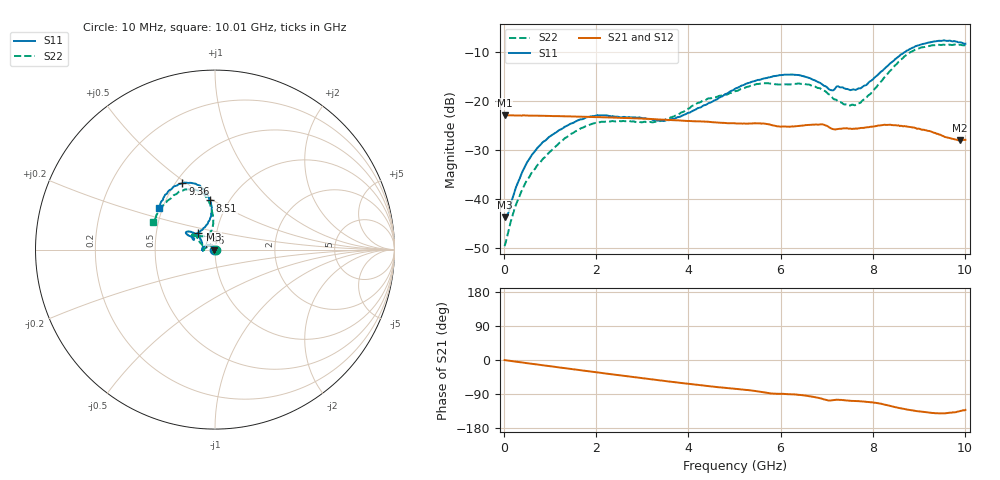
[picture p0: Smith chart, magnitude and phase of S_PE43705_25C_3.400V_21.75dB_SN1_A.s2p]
! Device ID: PE43705
! Serial: 1
! Insertion: A
! Impedance: 50 ohm
! Temp: 25C
! VDD: 3.400V
! Attenuation Step: 21.75dB
#  Hz  S  RI  R  50
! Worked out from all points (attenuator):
!   401 points, 10 MHz to 10.01 GHz, reference 50 ohm
!   highest |S21| = -22.82 dB at 10 MHz (marker M1); lowest = -28.0 dB at 9.885 GHz (marker M2)
!   lowest |S11| = -43.7 dB at 10 MHz (marker M3), VSWR 1.01, Z = 49.4 + j0.0459 ohm
!   |S11| at or under -10 dB: start of sweep to 8.682 GHz
!   |S22| runs from -49.6 to -8.4 dB; largest |S21 - S12| = 0.00086
!   S11 on the Smith chart (normalised r, x): 10 MHz: 0.99, +0.00; 7.46 GHz: 0.81, +0.16; 8.51 GHz: 0.82, +0.48; 9.36 GHz: 0.54, +0.48; 10.01 GHz: 0.48, +0.26
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1e7  -0.00652 0.000465  0.0723 -0.00027  0.0724 -0.000273  0.0033 0.000354
8.5e7  -0.00623 0.0035  0.0721 -0.00192  0.072 -0.00186  0.00364 0.00266
2.6e8  -0.00781 0.0109  0.0717 -0.00562  0.0716 -0.00552  0.00191 0.00869
5.85e8  -0.0165 0.0222  0.0705 -0.0121  0.0704 -0.0121  -0.00626 0.0172
1.01e9  -0.0356 0.0266  0.0679 -0.0204  0.068 -0.0203  -0.0246 0.0188
1.685e9  -0.0636 0.0161  0.0619 -0.0321  0.062 -0.032  -0.0528 0.00883
2.185e9  -0.0718 0.00183  0.0561 -0.0398  0.0561 -0.0397  -0.0618 -0.00126
3.36e9  -0.0635 0.00264  0.0387 -0.0527  0.0388 -0.0526  -0.0616 0.00885
3.86e9  -0.0669 0.0253  0.0309 -0.0556  0.0311 -0.0555  -0.0726 0.0269
5.01e9  -0.104 0.0853  0.0144 -0.0579  0.0145 -0.058  -0.1041 0.0731
5.535e9  -0.1336 0.0981  0.00672 -0.0592  0.00683 -0.0591  -0.1217 0.0894
6.01e9  -0.157 0.0994  0.000822 -0.0551  0.00114 -0.0552  -0.1199 0.0886
6.685e9  -0.1481 0.0789  -0.00706 -0.0573  -0.00688 -0.0574  -0.12 0.08
7.085e9  -0.1153 0.0612  -0.0154 -0.0511  -0.0153 -0.0512  -0.0846 0.078
7.46e9  -0.0943 0.0944  -0.0156 -0.0506  -0.0155 -0.0506  -0.0481 0.079
7.785e9  -0.0515 0.132  -0.0179 -0.0505  -0.0175 -0.0504  -0.024 0.1002
8.36e9  -0.0182 0.2393  -0.0295 -0.0495  -0.0292 -0.0495  -0.0142 0.2012
8.51e9  -0.0273 0.274  -0.0326 -0.0466  -0.0322 -0.0469  -0.0232 0.2374
8.91e9  -0.0813 0.3533  -0.0374 -0.0388  -0.0369 -0.0387  -0.0858 0.3249
9.36e9  -0.1815 0.3686  -0.0367 -0.0302  -0.0365 -0.0301  -0.184 0.3272
9.885e9  -0.2967 0.2717  -0.0282 -0.0283  -0.0286 -0.0282  -0.3195 0.2032
1.001e10  -0.3141 0.2297  -0.027 -0.0302  -0.0274 -0.0303  -0.3444 0.1522
